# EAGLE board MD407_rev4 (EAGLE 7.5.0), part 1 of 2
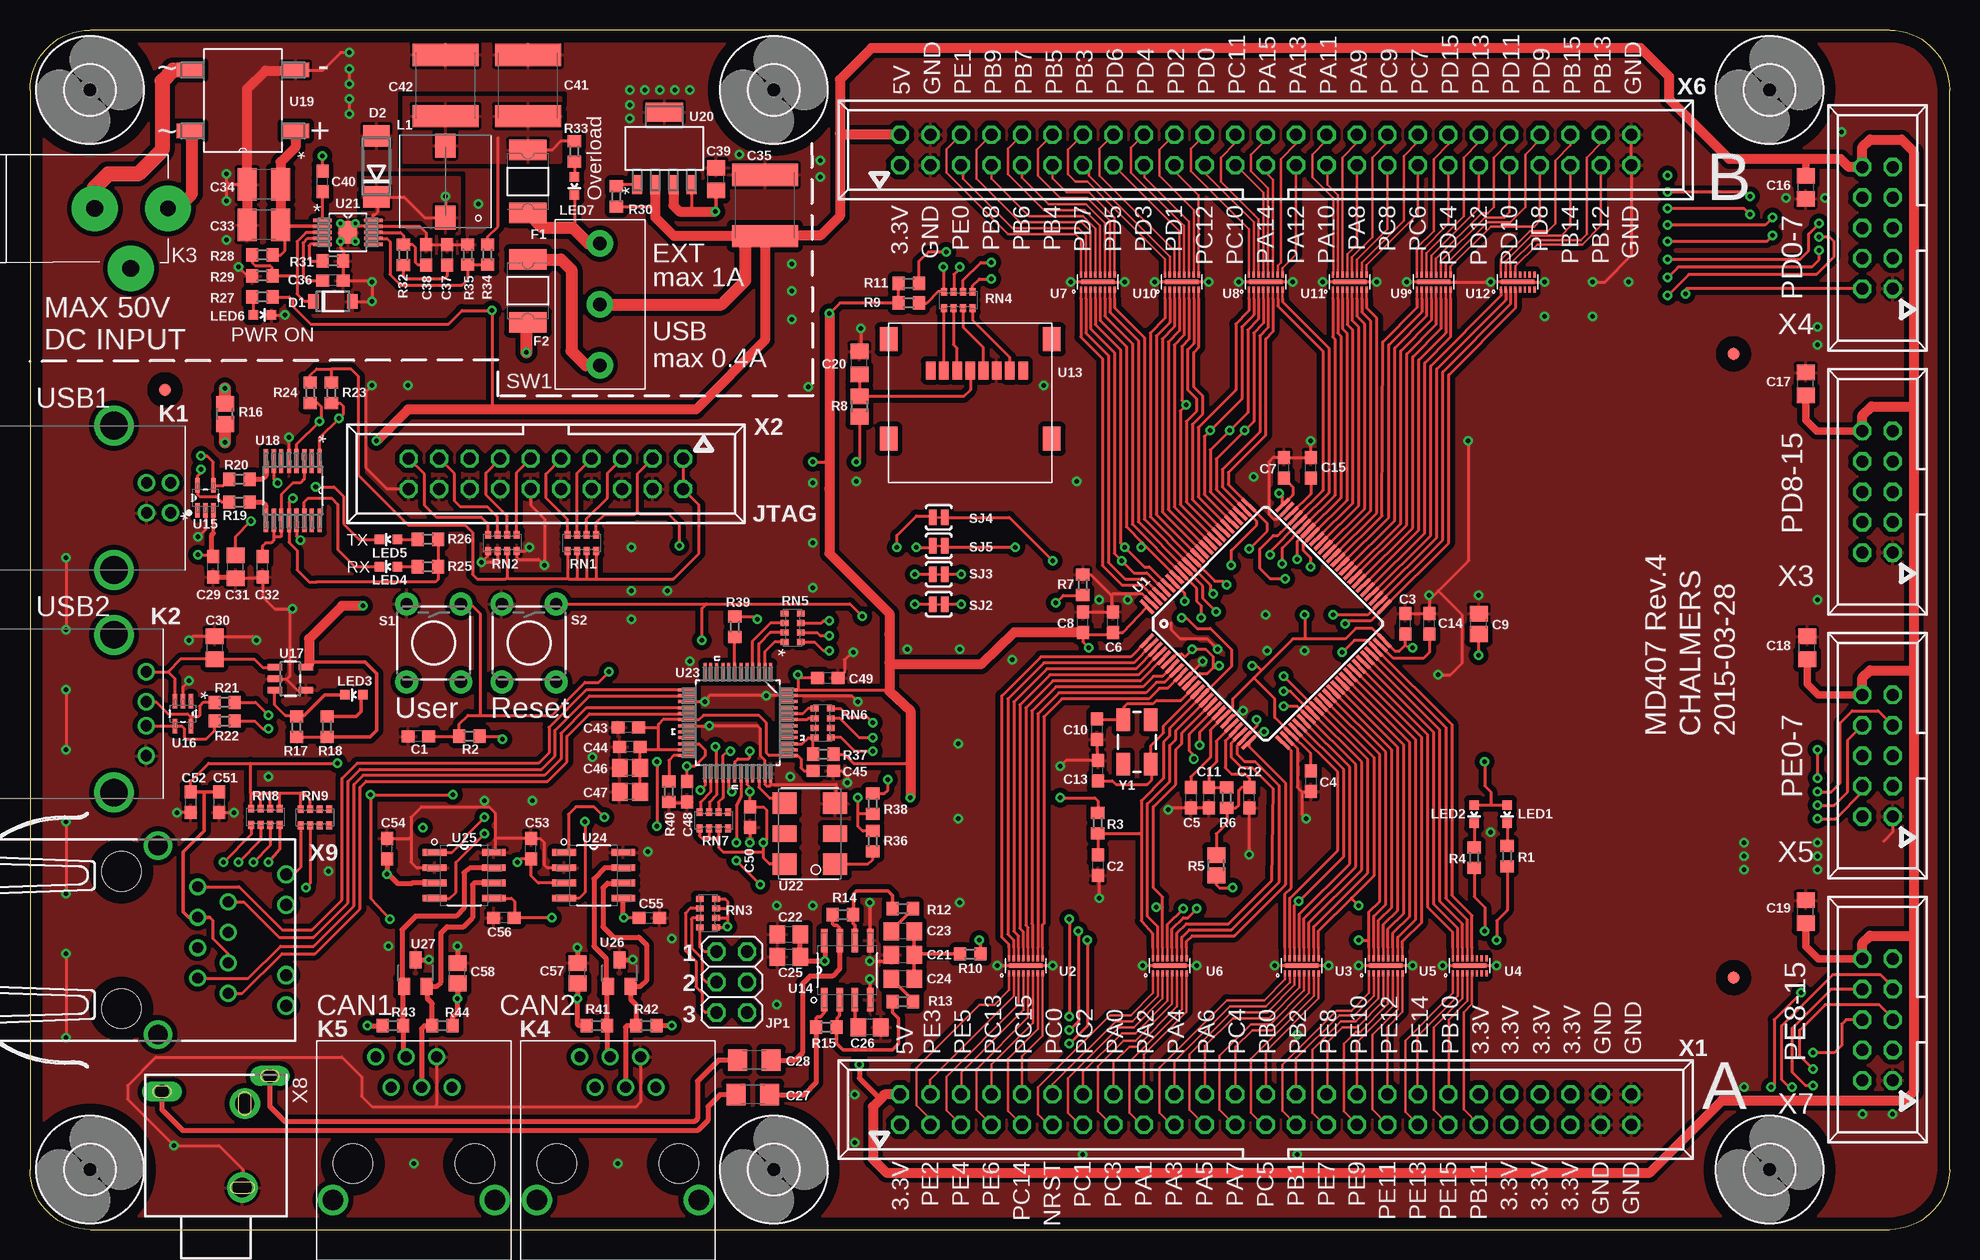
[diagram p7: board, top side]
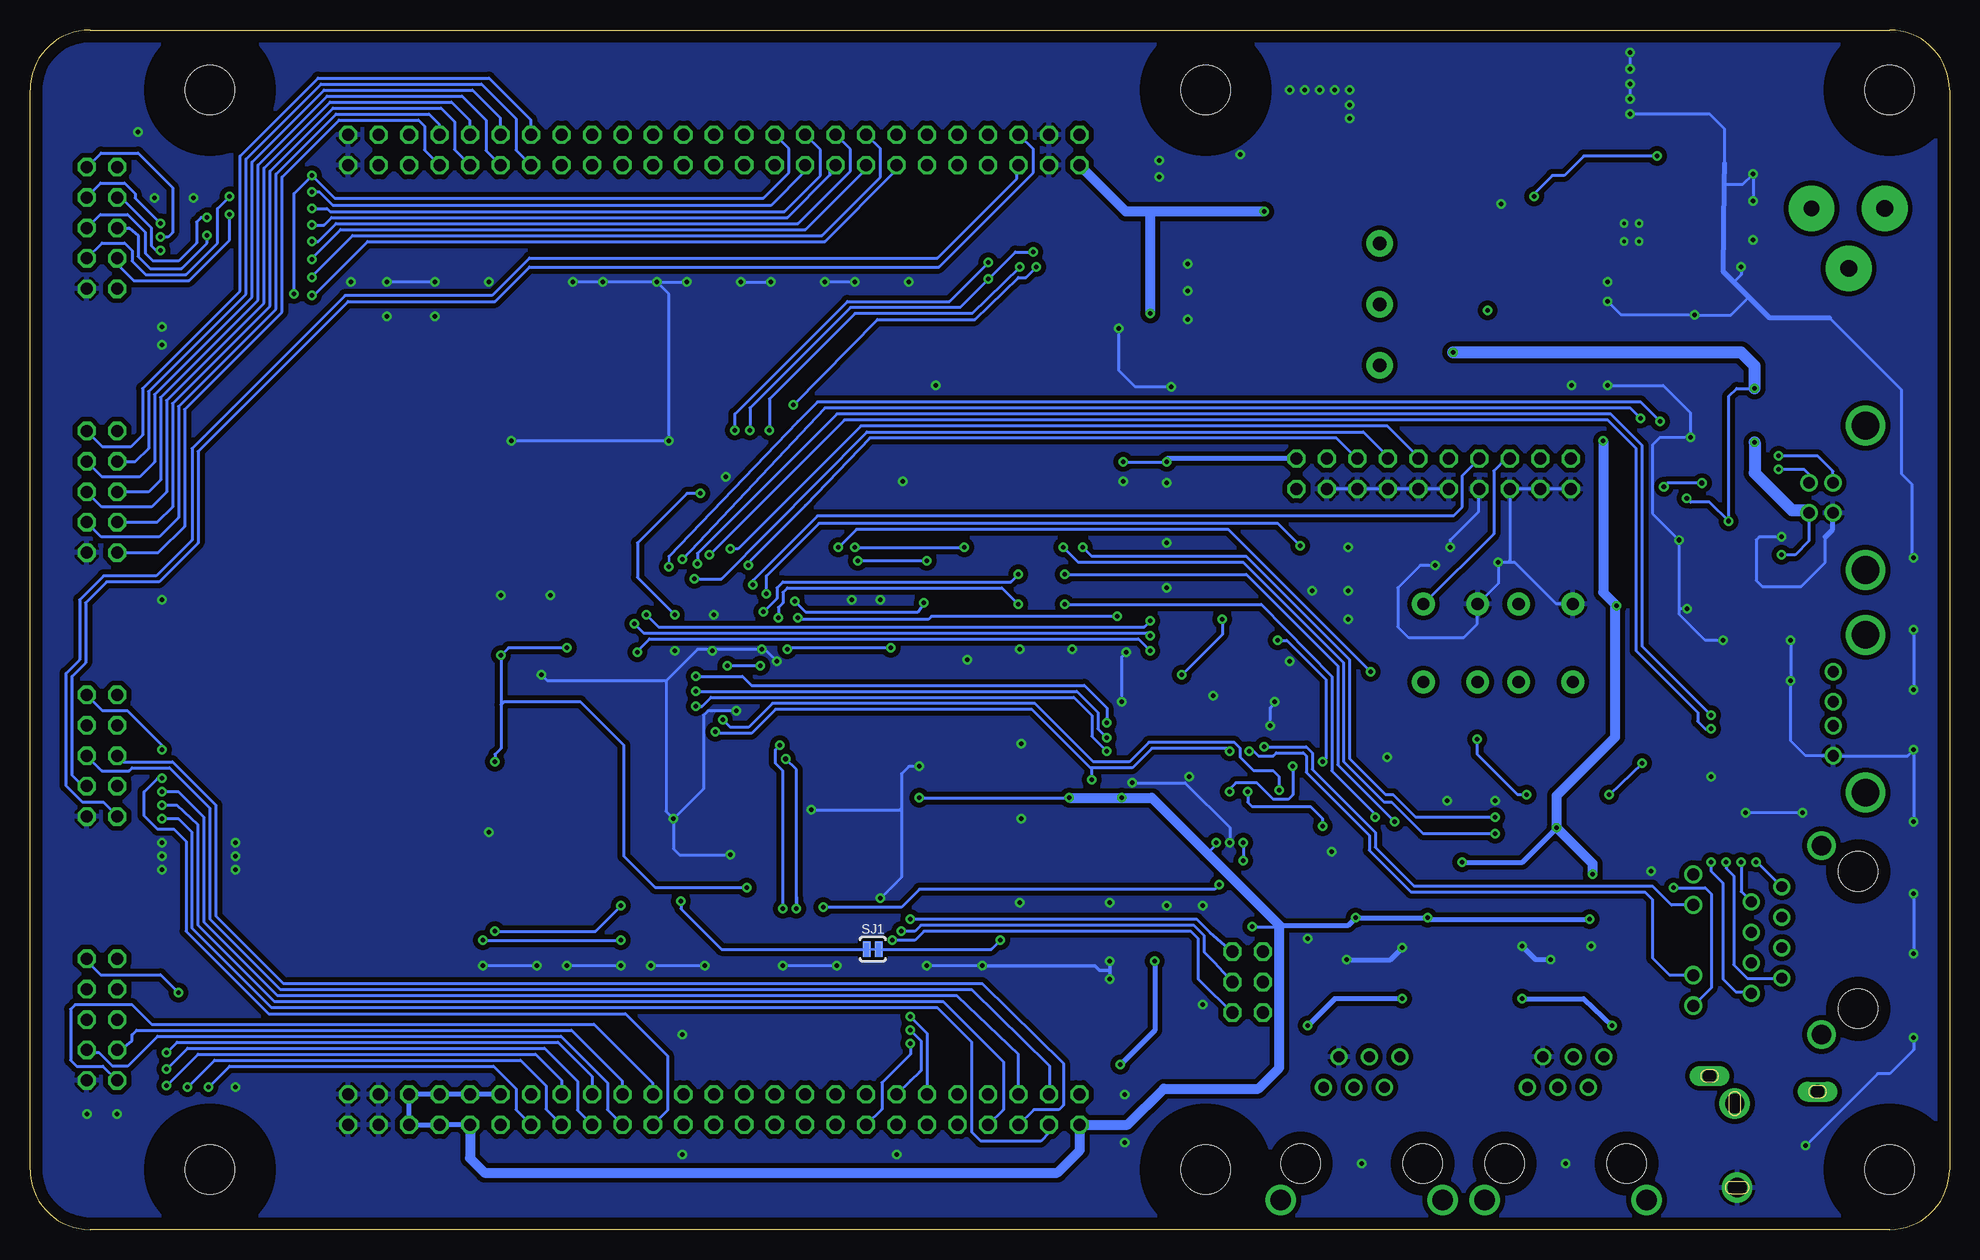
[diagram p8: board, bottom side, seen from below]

Size 160 x 100 mm. Coordinates in mm from the lower left corner, seen from the top.
Outline: 5,0 155,0 arc90 160,5 160,95 arc90 155,100 5,100 arc90 0,95 0,5 arc90 5,0
Copper layers (1*16): Top 0.035mm / dielectric 1.5mm / Bottom 0.035mm
Design rules "default *": minimum track width 0.2mm, minimum drill 0.3mm, track to track 5mil, track to pad 3mil, pad to pad 3mil, via to via 8mil, smd to smd 4mil, copper to edge 40mil, drill to drill 8mil, minimum pad ring 10mil, minimum via ring 8mil, stop-mask expansion 1mil, vias tented up to drill 16mil, thermal gap 10mil
Net classes: 1 HP: width 0.762 mm

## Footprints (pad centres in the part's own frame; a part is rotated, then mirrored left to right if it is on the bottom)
C0603 = smd 1.1 x 1: 1 -0.85,0; 2 0.85,0
C0805 = smd 1.3 x 1.5: 1 -0.85,0; 2 0.85,0
C0805' = smd 1.3 x 1.5: 1 -0.95,0; 2 0.95,0
C1206 = smd 1.6 x 1.8: 1 -1.4,0; 2 1.4,0
C1210 = smd 1.6 x 2.7: 1 -1.4,0; 2 1.4,0
C2220K = smd 1.85 x 5.5: 1 -2.55,0; 2 2.55,0
SOD123FL = smd 0.91 x 1.22: A 1.625,0; C -1.625,0
DO214AA = smd 1.8 x 2.2: A 2.55,0; C -2.55,0
PTC1812L = smd 1.7 x 3.15: 1 -2.62,0; 2 2.62,0
4,1 = hole 4.1: 0,0
2X03 = drill 1.016 octagon: 1 -2.54,-1.27; 2 -2.54,1.27; 3 0,-1.27; 4 0,1.27; 5 2.54,-1.27; 6 2.54,1.27
61400416121 = drill 0.92: 1 1.25,4.71; 2 -1.25,4.71; 3 -1.25,2.71; 4 1.25,2.71 | drill 2.3: Z1 -6.02,0; Z2 6.02,0
61400416021 = drill 0.92: 1 -3.5,2.7; 2 -1,2.7; 3 1,2.7; 4 3.5,2.7 | drill 2.3: 5 -6.57,0; 6 6.57,0
DC-PLUG = drill 1.3 pad 3.81: 1 0,0 | drill 1.4 pad 3.81: 2 3.1,5; 3 6.1,0
615006143421 = drill 0.9: 1 -3.175,8.89; 2 -1.905,6.35; 3 -0.635,8.89; 4 0.635,6.35; 5 1.905,8.89; 6 3.175,6.35 | drill 1.7: Z1 -6.75,-3.05; Z2 6.75,-3.05 | hole 3.25: -5.08,0; 5.08,0
WE-PD_7332/7345_PLASTIC_BASE = smd 1.7 x 2: 1 0,3; 2 0,-3
LED-0603 = smd 0.8 x 0.8: A 0,-0.75; C 0,0.75
R0603 = smd 1 x 1.1: 1 -0.85,0; 2 0.85,0
R0805 = smd 1.3 x 1.5: 1 -0.85,0; 2 0.85,0
CAY16 = smd 0.5 x 0.65: 1 -1.2,-0.675; 2 -0.4,-0.675; 3 0.4,-0.675; 4 1.2,-0.675; 5 1.2,0.675; 6 0.4,0.675; 7 -0.4,0.675; 8 -1.2,0.675
TACTILE-PTH = drill 1.016 pad 1.88: 1 -3.251,2.261; 2 3.251,2.261; 3 -3.251,-2.261; 4 3.251,-2.261
SJ_2S-TRACE = smd 0.635 x 1.27: 1 -0.508,0; 2 0.508,0
25436N = drill 1.1 pad 2.184: P$1 0,-5.08; P$2 0,0; P$3 0,5.08
LQFP100 = smd 1.5 x 0.3: 1 -8,6; 2 -8,5.5; 3 -8,5; 4 -8,4.5; 5 -8,4; 6 -8,3.5; 7 -8,3; 8 -8,2.5; 9 -8,2; 10 -8,1.5; 11 -8,1; 12 -8,0.5; 13 -8,0; 14 -8,-0.5; 15 -8,-1; 16 -8,-1.5; 17 -8,-2; 18 -8,-2.5; 19 -8,-3; 20 -8,-3.5; 21 -8,-4; 22 -8,-4.5; 23 -8,-5; 24 -8,-5.5; 25 -8,-6; 51 8,-6; 52 8,-5.5; 53 8,-5; 54 8,-4.5; 55 8,-4; 56 8,-3.5; 57 8,-3; 58 8,-2.5; 59 8,-2; 60 8,-1.5; 61 8,-1; 62 8,-0.5; 63 8,0; 64 8,0.5; 65 8,1; 66 8,1.5; 67 8,2; 68 8,2.5; 70 8,3.5; 71 8,4; 72 8,4.5; 73 8,5; 74 8,5.5; 75 8,6 | smd 0.3 x 1.5: 26 -6,-8; 27 -5.5,-8; 28 -5,-8; 29 -4.5,-8; 30 -4,-8; 31 -3.5,-8; 32 -3,-8; 33 -2.5,-8; 34 -2,-8; 35 -1.5,-8; 36 -1,-8; 37 -0.5,-8; 38 0,-8; 39 0.5,-8; 40 1,-8; 41 1.5,-8; 42 2,-8; 43 2.5,-8; 44 3,-8; 45 3.5,-8; 46 4,-8; 47 4.5,-8; 48 5,-8; 49 5.5,-8; 50 6,-8; 76 6,8; 77 5.5,8; 78 5,8; 79 4.5,8; 80 4,8; 81 3.5,8; 82 3,8; 83 2.5,8; 84 2,8; 85 1.5,8; 86 1,8; 87 0.5,8; 88 0,8; 89 -0.5,8; 90 -1,8; 91 -1.5,8; 92 -2,8; 93 -2.5,8; 94 -3,8; 95 -3.5,8; 96 -4,8; 97 -4.5,8; 98 -5,8; 99 -5.5,8; 100 -6,8 | smd 1.5 x 0.35: 69 8,3
16-WFDFN = smd 0.2 x 0.5: 1 -1.4,-0.625; 2 -1,-0.625; 3 -0.6,-0.625; 4 -0.2,-0.625; 5 0.2,-0.625; 6 0.6,-0.625; 7 1,-0.625; 8 1.4,-0.625; 9 1.4,0.625; 10 1,0.625; 11 0.6,0.625; 12 0.2,0.625; 13 -0.2,0.625; 14 -0.6,0.625; 15 -1,0.625; 16 -1.4,0.625 | smd 2.8 x 0.4: 17 0,0
MICROSD_500901-0801 = smd 0.8 x 1.5: P$1 -3.3,0.75; P$2 -2.2,0.75; P$3 -1.1,0.75; P$4 0,0.75; P$5 1.1,0.75; P$6 2.2,0.75; P$7 3.3,0.75; P$8 4.4,0.75 | smd 1.45 x 2: P$9 -6.8,3.35; P$10 6.8,3.35; P$11 -6.8,-4.95; P$12 6.8,-4.95
SOIC127P600X175-8N = smd 1.981 x 0.559: 1 -2.464,1.905; 2 -2.464,0.635; 3 -2.464,-0.635; 4 -2.464,-1.905; 5 2.464,-1.905; 6 2.464,-0.635; 7 2.464,0.635; 8 2.464,1.905
SOT65P220X110-5N = smd 1.168 x 0.356: 1 -1.041,0.66; 2 -1.041,0; 3 -1.041,-0.66; 4 1.041,-0.66; 5 1.041,0.66
SOT23-5 = smd 0.55 x 1.2: 1 -0.95,-1.3; 2 0,-1.3; 3 0.95,-1.3; 4 0.95,1.3; 5 -0.95,1.3
SOP63P600X175-16N = smd 1.981 x 0.356: 1 -2.464,2.235; 2 -2.464,1.575; 3 -2.464,0.965; 4 -2.464,0.305; 5 -2.464,-0.305; 6 -2.464,-0.965; 7 -2.464,-1.575; 8 -2.464,-2.235; 9 2.464,-2.235; 10 2.464,-1.575; 11 2.464,-0.965; 12 2.464,-0.305; 13 2.464,0.305; 14 2.464,0.965; 15 2.464,1.575; 16 2.464,2.235
SOT508P985X260-4N = smd 2.235 x 1.245: 1 -4.394,2.54; 2 -4.394,-2.54; 3 4.394,-2.54; 4 4.394,2.54
SOT15P696X180-5N = smd 1.6 x 0.838: 1 -3.023,2.261; 2 -3.023,0.762; 3 -3.023,-0.762; 4 -3.023,-2.261 | smd 1.6 x 3.099: 5 3.023,0
SOP50P490X110-11N = smd 1.549 x 0.279: 1 -2.108,0.991; 2 -2.108,0.508; 3 -2.108,0; 4 -2.108,-0.508; 5 -2.108,-0.991; 6 2.108,-0.991; 7 2.108,-0.508; 8 2.108,0; 9 2.108,0.508; 10 2.108,0.991 | smd 1.575 x 1.88: 11 0,0
CRYSTAL-SMD-7.5X5.2-6PIN = smd 1.8 x 2: 1 -2.54,-2.1; 2 2.54,-2.1; 3 2.54,2.1; 4 -2.54,2.1 | smd 1.4 x 2: NC0 0,-2.1; NC1 0,2.1
QFP50P900X900X160-48N = smd 1.473 x 0.254: 1 -4.242,2.743; 2 -4.242,2.261; 3 -4.242,1.753; 4 -4.242,1.245; 5 -4.242,0.762; 6 -4.242,0.254; 7 -4.242,-0.254; 8 -4.242,-0.762; 9 -4.242,-1.245; 10 -4.242,-1.753; 11 -4.242,-2.261; 12 -4.242,-2.743; 25 4.242,-2.743; 26 4.242,-2.261; 27 4.242,-1.753; 28 4.242,-1.245; 29 4.242,-0.762; 30 4.242,-0.254; 31 4.242,0.254; 32 4.242,0.762; 33 4.242,1.245; 34 4.242,1.753; 35 4.242,2.261; 36 4.242,2.743 | smd 0.254 x 1.473: 13 -2.743,-4.242; 14 -2.261,-4.242; 15 -1.753,-4.242; 16 -1.245,-4.242; 17 -0.762,-4.242; 18 -0.254,-4.242; 19 0.254,-4.242; 20 0.762,-4.242; 21 1.245,-4.242; 22 1.753,-4.242; 23 2.261,-4.242; 24 2.743,-4.242; 37 2.743,4.242; 38 2.261,4.242; 39 1.753,4.242; 40 1.245,4.242; 41 0.762,4.242; 42 0.254,4.242; 43 -0.254,4.242; 44 -0.762,4.242; 45 -1.245,4.242; 46 -1.753,4.242; 47 -2.261,4.242; 48 -2.743,4.242
SOT23 = smd 1 x 1.4: 1 -0.95,-1.1; 2 0.95,-1.1; 3 0,1.1
FIDUCIAL_1MM = smd 1 x 1: 1 0,0
057-050-1 = drill 1 octagon: 1 -30.48,-1.27; 2 -30.48,1.27; 3 -27.94,-1.27; 4 -27.94,1.27; 5 -25.4,-1.27; 6 -25.4,1.27; 7 -22.86,-1.27; 8 -22.86,1.27; 9 -20.32,-1.27; 10 -20.32,1.27; 11 -17.78,-1.27; 12 -17.78,1.27; 13 -15.24,-1.27; 14 -15.24,1.27; 15 -12.7,-1.27; 16 -12.7,1.27; 17 -10.16,-1.27; 18 -10.16,1.27; 19 -7.62,-1.27; 20 -7.62,1.27; 21 -5.08,-1.27; 22 -5.08,1.27; 23 -2.54,-1.27; 24 -2.54,1.27; 25 0,-1.27; 26 0,1.27; 27 2.54,-1.27; 28 2.54,1.27; 29 5.08,-1.27; 30 5.08,1.27; 31 7.62,-1.27; 32 7.62,1.27; 33 10.16,-1.27; 34 10.16,1.27; 35 12.7,-1.27; 36 12.7,1.27; 37 15.24,-1.27; 38 15.24,1.27; 39 17.78,-1.27; 40 17.78,1.27; 41 20.32,-1.27; 42 20.32,1.27; 43 22.86,-1.27; 44 22.86,1.27; 45 25.4,-1.27; 46 25.4,1.27; 47 27.94,-1.27; 48 27.94,1.27; 49 30.48,-1.27; 50 30.48,1.27
057-020-1 = drill 1 octagon: 1 -11.43,-1.27; 2 -11.43,1.27; 3 -8.89,-1.27; 4 -8.89,1.27; 5 -6.35,-1.27; 6 -6.35,1.27; 7 -3.81,-1.27; 8 -3.81,1.27; 9 -1.27,-1.27; 10 -1.27,1.27; 11 1.27,-1.27; 12 1.27,1.27; 13 3.81,-1.27; 14 3.81,1.27; 15 6.35,-1.27; 16 6.35,1.27; 17 8.89,-1.27; 18 8.89,1.27; 19 11.43,-1.27; 20 11.43,1.27
057-010-1 = drill 1 octagon: 1 -5.08,-1.27; 2 -5.08,1.27; 3 -2.54,-1.27; 4 -2.54,1.27; 5 0,-1.27; 6 0,1.27; 7 2.54,-1.27; 8 2.54,1.27; 9 5.08,-1.27; 10 5.08,1.27
KLBR4 = drill 1.6 pad 2.54: B -2.4,-3.5; S -2.2,3.5 | drill 1.1 pad 1.2 long: R -4.5,-5.8; T 4.5,-4.5
J1 = drill 0.9 pad 1.3: 1 4.445,2.54; 2 3.175,0; 3 1.905,2.54; 4 0.635,0; 5 -0.635,2.54; 6 -1.905,0; 7 -3.175,2.54; 8 -4.445,0 | drill 1 pad 1.422: 9 5.465,7.37; 10 2.925,7.37; 11 -2.925,7.37; 12 -5.465,7.37 | drill 1.6 pad 2.184: M1 -7.875,-3.3; M2 7.875,-3.3 | hole 3.3: 5.715,-6.35; -5.715,-6.35
CRYSTAL-SMD-5X3 = smd 1.9 x 1.1: 1 -1.85,-1.15; 2 1.85,-1.15; 3 1.85,1.15; 4 -1.85,1.15

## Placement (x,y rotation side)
C1  100n  [C0603]  32.38,41.12 180 top
C2  100n  [C0603]  89,30.38 270 top
C3  100n  [C0603]  114.62,50.5 90 top
C4  100n  [C0603]  106.75,37.38 270 top
C5  100n  [C0603]  96.75,36 270 top
C6  100n  [C0603]  90.25,50.62 90 top
C7  100n  [C0603]  104.5,63.5 90 top
C8  100n  [C0603]  87.75,50.62 90 top
C9  4u7/X7R/16V  [C0805]  120.75,50.5 90 top
C10  22p  [C0603]  88.96,41.72 90 top
C11  2u2/X5R/6V3  [C0603]  98.25,36 270 top
C12  2u2/X5R/6V3  [C0603]  101.62,36 90 top
C13  22p  [C0603]  89,38.25 90 top
C14  2u2/X5R/6V3  [C0603]  116.62,50.5 90 top
C15  2u2/X5R/6V3  [C0603]  106.75,63.5 90 top
C16  4u7/X7R/16V  [C0805']  148,86.88 270 top
C17  4u7/X7R/16V  [C0805']  148,70.5 90 top
C18  4u7/X7R/16V  [C0805']  148.12,48.5 90 top
C19  4u7/X7R/16V  [C0805']  148,26.5 90 top
C20  4u7/X7R/16V  [C0805']  69.12,72.25 90 top
C21  220n/X7R/25V  [C0805']  72.75,22.91 180 top
C22  4u7/X7R/16V  [C0805']  63.25,24.62 0 top
C23  1u/X7R/25V  [C0805']  72.75,24.88 180 top
C24  1u/X7R/25V  [C0805']  72.75,20.91 180 top
C25  4u7/X7R/16V  [C0805']  63.25,22.75 0 top
C26  1u/X7R/25V  [C0805']  69.98,16.87 180 top
C27  22u/X5R/6V3  [C1206]  60.25,11.25 180 top
C28  22u/X5R/6V3  [C1206]  60.38,14.12 180 top
C29  100n  [C0603]  15.25,55.25 90 top
C30  4u7/X7R/16V  [C0805']  15.38,48.5 270 top
C31  4u7/X7R/16V  [C0805']  17.12,55.25 90 top
C32  100n  [C0603]  19.38,55.25 90 top
C33  4u7/X7S/100V  [C1210]  19.5,83.75 180 top
C34  4u7/X7S/100V  [C1210]  19.5,87.12 180 top
C35  47u/X7R/16V  [C2220K]  61.25,85.38 90 top
C36  3n9  [C0603]  25.25,79.12 180 top
C37  2n7  [C0603]  34.75,81.25 270 top
C38  4p7  [C0603]  33,81.25 270 top
C39  4u7/X7R/16V  [C0805']  57.19,87.57 90 top
C40  100n  [C0603]  24.38,87.38 90 top
C41  47u/X7R/16V  [C2220K]  41.5,95.38 90 top
C42  47u/X7R/16V  [C2220K]  34.62,95.38 90 top
C43  100n  [C0603]  49.88,41.88 180 top
C44  100n  [C0603]  50,40.25 180 top
C45  100n  [C0603]  66.12,38.25 0 top
C46  4u7/X7R/16V  [C0805]  50,38.5 180 top
C47  4u7/X7R/16V  [C0805]  50,36.5 180 top
C48  100n  [C0603]  54.75,36.5 270 top
C49  100n  [C0603]  66.5,46 0 top
C50  100n  [C0603]  60,34.38 270 top
C51  100n  [C0603]  15.75,35.62 270 top
C52  100n  [C0603]  13.38,35.62 270 top
C53  100n  [C0603]  41.75,31.75 90 top
C54  100n  [C0603]  29.75,31.75 90 top
C55  100n  [C0603]  51.62,26 0 top
C56  100n  [C0603]  39.5,26 180 top
C57  4.7nF/100V  [C0805]  45.62,21.38 90 top
C58  4.7nF/100V  [C0805]  35.62,21.38 90 top
D1  SMF5.0AT1  [SOD123FL]  25.25,77.38 0 top
D2  SS2H10-E3/52T  [DO214AA]  28.88,88.62 90 top
F1  1A  [PTC1812L]  41.5,87.38 90 top
F2  400mA  [PTC1812L]  41.5,78.25 270 top
H1  MOUNT-HOLE4.1  [4,1]  145,5 0 top
H2  MOUNT-HOLE4.1  [4,1]  5,5 0 top
H3  MOUNT-HOLE4.1  [4,1]  62,5 0 top
H4  MOUNT-HOLE4.1  [4,1]  5,95 0 top
H5  MOUNT-HOLE4.1  [4,1]  62,95 0 top
H6  MOUNT-HOLE4.1  [4,1]  145,95 0 top
JP1  [2X03]  58.5,20.62 270 top
K1  61400416121  [61400416121]  7,61 270 top
K2  61400416021  [61400416021]  7,43 270 top
K3  FC681465P  [DC-PLUG]  11.5,85.12 180 top
K4  615006143421  [615006143421]  49,5.5 0 top
K5  615006143421  [615006143421]  32,5.5 0 top
L1  7447789118  [WE-PD_7332/7345_PLASTIC_BASE]  34.62,87.38 180 top
LED1  RED  [LED-0603]  123.12,34.62 180 top
LED2  Green  [LED-0603]  120.38,34.62 180 top
LED3  RED  [LED-0603]  27,44.58 90 top
LED4  Green  [LED-0603]  29.86,55.26 90 top
LED5  Blue  [LED-0603]  29.86,57.54 90 top
LED6  Green  [LED-0603]  19.38,76.25 270 top
LED7  RED  [LED-0603]  45.38,87 180 top
R1  100R  [R0603]  123.12,31.12 90 top
R2  10k  [R0603]  36.62,41.12 0 top
R3  10k  [R0603]  89,33.88 90 top
R4  100R  [R0603]  120.38,31 90 top
R5  742792097  [R0805]  98.88,30.38 90 top
R6  59R  [R0603]  99.75,36 270 top
R7  75k  [R0603]  87.75,53.75 270 top
R8  742792097  [R0805]  69.12,68.62 270 top
R9  10k  [R0603]  73.25,77.25 180 top
R10  27R  [R0603]  78.38,22.97 180 top
R11  10k  [R0603]  73.25,78.88 180 top
R12  20k  [R0603]  72.75,26.75 180 top
R13  20k  [R0603]  72.75,19 180 top
R14  20k  [R0603]  67.75,26.25 180 top
R15  20k  [R0603]  66.38,16.88 180 top
R16  742792097  [R0805]  16.25,68 90 top
R17  30k  [R0603]  22.23,41.91 270 top
R18  620R  [R0603]  24.77,41.91 270 top
R19  27R  [R0603]  17.44,60.64 180 top
R20  27R  [R0603]  17.44,62.55 180 top
R21  27R  [R0603]  16.23,43.95 180 top
R22  27R  [R0603]  16.23,42.39 180 top
R23  10k  [R0603]  25.12,69.75 90 top
R24  10k  [R0603]  23.36,69.77 90 top
R25  620R  [R0603]  33.16,55.26 0 top
R26  620R  [R0603]  33.16,57.54 0 top
R27  620R  [R0603]  19.38,77.75 0 top
R28  dnm  [R0603]  19.38,81.25 0 top
R29  dnm  [R0603]  19.38,79.5 0 top
R30  10k  [R0603]  48.88,86.12 270 top
R31  200k  [R0603]  25.25,80.75 180 top
R32  75k  [R0603]  31.12,81.25 90 top
R33  620R  [R0603]  45.38,89.88 270 top
R34  30k  [R0603]  38.14,81.28 90 top
R35  5k6  [R0603]  36.49,81.28 270 top
R36  2k2  [R0603]  70.25,32.38 90 top
R37  1k5  [R0603]  66.12,39.62 180 top
R38  1k5  [R0603]  70.25,35.5 90 top
R39  2k2  [R0603]  58.75,50.25 270 top
R40  4.87k  [R0603]  53.25,36.5 90 top
R41  59R  [R0603]  47.25,17 0 top
R42  59R  [R0603]  51.38,17 0 top
R43  59R  [R0603]  30.25,17 0 top
R44  59R  [R0603]  34.38,17 0 top
RN1  10k  [CAY16]  46,57.25 180 top
RN2  10k  [CAY16]  39.38,57.25 180 top
RN3  10k  [CAY16]  56.5,26.38 90 top
RN4  27R  [CAY16]  77.38,77.5 0 top
RN5  51R  [CAY16]  63.58,50.17 90 top
RN6  51R  [CAY16]  66.08,42.23 90 top
RN7  2k2  [CAY16]  57,34.12 180 top
RN8  51R  [CAY16]  19.62,34.41 180 top
RN9  330R  [CAY16]  23.75,34.38 0 top
S1  SKQBARA010PTH  [TACTILE-PTH]  33.66,48.9 270 top
S2  SKQBARA010PTH  [TACTILE-PTH]  41.59,48.9 270 top
SJ1  SOLDERJUMPERTRACE  [SJ_2S-TRACE]  89.75,23.38 0 bottom
SJ2  SOLDERJUMPERTRACE  [SJ_2S-TRACE]  75.75,52.12 180 top
SJ3  SOLDERJUMPERTRACE  [SJ_2S-TRACE]  75.75,54.62 180 top
SJ4  SOLDERJUMPERTRACE  [SJ_2S-TRACE]  75.75,59.38 180 top
SJ5  SOLDERJUMPERTRACE  [SJ_2S-TRACE]  75.75,57 180 top
SW1  25436NAH  [25436N]  47.5,77.12 0 top
U1  STM32F407VGT7  [LQFP100]  103,50.5 45 top
U2  TPD8F003  [16-WFDFN]  83,22 0 top
U3  TPD8F003  [16-WFDFN]  106,22 0 top
U4  TPD8F003  [16-WFDFN]  120,22 0 top
U5  TPD8F003  [16-WFDFN]  113,22 0 top
U6  TPD8F003  [16-WFDFN]  95,22 0 top
U7  TPD8F003  [16-WFDFN]  89,79 0 top
U8  TPD8F003  [16-WFDFN]  103,79 0 top
U9  TPD8F003  [16-WFDFN]  117,79 0 top
U10  TPD8F003  [16-WFDFN]  96,79 0 top
U11  TPD8F003  [16-WFDFN]  110,79 0 top
U12  TPD8F003  [16-WFDFN]  124,79 0 top
U13  500901-0801  [MICROSD_500901-0801]  78.38,70.88 0 top
U14  TPA6111A2D  [SOIC127P600X175-8N]  68.12,21.62 90 top
U15  SP3003-02JTG  [SOT65P220X110-5N]  14.62,61 90 top
U16  SP3003-02JTG  [SOT65P220X110-5N]  12.75,43 270 top
U17  STMPS2141STR  [SOT23-5]  21.71,45.91 270 top
U18  FT230XS  [SOP63P600X175-16N]  21.91,61.59 270 top
U19  DF01S  [SOT508P985X260-4N]  17.75,94.12 180 top
U20  LP3875EMP-3.3  [SOT15P696X180-5N]  52.88,90.12 90 top
U21  TPS54160ADGQ  [SOP50P490X110-11N]  26.5,83.12 0 top
U22  FXO-HC736R-50  [CRYSTAL-SMD-7.5X5.2-6PIN]  65,33 90 top
U23  DP83848CVV  [QFP50P900X900X160-48N]  59,42.25 270 top
U24  MAX13054ASA+  [SOIC127P600X175-8N]  46.99,29.53 0 top
U25  MAX13054ASA+  [SOIC127P600X175-8N]  36.2,29.53 0 top
U26  PESD2CAN,215  [SOT23]  49.12,21.38 0 top
U27  PESD2CAN,215  [SOT23]  32.12,21.38 0 top
U$1  FIDUCIAL  [FIDUCIAL_1MM]  11.25,70 0 top
U$2  FIDUCIAL  [FIDUCIAL_1MM]  142,21 0 top
U$3  FIDUCIAL  [FIDUCIAL_1MM]  142,73 0 top
U$4  [A4L-LOC]  not placed on the board
X1  61205021621  [057-050-1]  103,10 0 top
X2  61202021621  [057-020-1]  43,63 180 top
X3  61201021621  [057-010-1]  154,61.5 90 top
X4  61201021621  [057-010-1]  154,83.5 90 top
X5  61201021621  [057-010-1]  154,39.5 90 top
X6  61205021621  [057-050-1]  103,90 0 top
X7  61201021621  [057-010-1]  154,17.5 90 top
X8  KLBR4  [KLBR4]  15.5,7 180 top
X9  J1011F01PNL  [J1]  13.97,24.13 270 top
Y1  8MHz  [CRYSTAL-SMD-5X3]  92.27,40.65 90 top

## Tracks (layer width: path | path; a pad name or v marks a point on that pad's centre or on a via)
3.3V  (via drill 0.4)
  Top 0.254: X9.3 16.51,22.99 15.25,24.25 15.25,25.75 14.96,26.04 X9.6 | 20,36.38 19.25,36.38 | 19.25,36.38 18.38,36.38 | RN8.3 19.23,36.35 19.25,36.38 | RN8.2 20.02,36.35 20,36.38 | 93.09,51.91 U1.100 91.09,49.77 C6.1 90.22,49.62 87.78,49.62 C8.1 87.75,49 v88.25,48.5 | 114.62,48.75 114.12,48.25 113.75,48.25 112.91,49.09 | 114.62,48.75 C3.1 | 96.64,45.51 U1.11 96.67,45.55 97.5,46.38 98.12,46.38 98.62,46.88 | U1.75 104.41,60.41 | C7.1 105.25,61.9 105.25,61.23 U1.75 | U1.6 94.88,47.32 95.56,48 96,48 96.25,47.75 v96.88,48.38 98,48.38 98.62,47.75 98.62,46.88 | U1.75 104.41,61.09 v104.12,61.38 | C4.1 106.75,39.68 U1.28 105.06,41.37 103.75,42.69 103.75,44.25 102,46 | U23.48 64,44.99 | 64,44.99 71.51,44.99 71.62,44.88 | R39.1 60.4,51.1 v60.62,50.88 | 64,44.99 v64,46.25 64.25,46 C49.1 | 22.5,36.38 22.88,36.38 23.35,35.9 RN9.7 | 22.5,36.38 20.88,36.38 | 20.88,36.38 20,36.38 | 22.5,36.38 22.55,36.33 RN9.8 | RN8.4 18.43,36.33 18.38,36.38 | RN8.1 20.82,36.33 20.88,36.38 | RN7.5 55.8,32.83 56,32.62 56.62,32.62 | 56.62,32.62 57.25,32.62 57.4,32.77 RN7.7 57.4,31.85 57.75,31.5 61.12,31.5 | RN7.6 56.6,32.65 56.62,32.62 | U23.22 55.75,40.5 56.25,40 56.25,39.5 55.38,38.62 v54.75,38.62 C48.1 | 71.65,49.65 71.62,49.62 | 18.38,38.88 14.88,38.88 13.38,37.38 C52.1 | 18.38,38.88 v25.62,38.88 | v30,25.88 28.38,27.62 v28.38,36.25 v35.25,36.25 | 112.91,49.09 111.88,50.12 110.5,50.12 109.62,49.25 106.25,49.25 | 106.25,49.25 105.25,49.25 102.62,46.62 | 102.62,46.62 102,46 | v106.25,51.25 106.25,49.25 | U1.50 112.91,49.09 | 98.62,46.88 99,46.88 v99.12,47 | v101.88,47 102.25,47 102.62,46.62 | v115.25,48.5 114.75,48.62 114.62,48.75 | 25.12,71.75 23.88,71.75 23.36,71.23 R24.2
  Top 0.254: 44.88,54.25 45.5,54.25 | 45.5,54.25 46.38,54.25 | 46.38,54.25 47.12,54.25 | RN1.5 44.8,54.33 44.88,54.25 | RN1.6 45.6,54.35 45.5,54.25 | RN1.7 46.4,54.27 46.38,54.25 | 47.12,54.25 47.2,54.33 RN1.8 | R23.2 25.12,71.75 | 25.12,71.75 26.75,71.75 27.38,71.12 27.38,62.88 31.5,58.75 36.25,58.75 36.88,58.12 36.88,54.62 37.25,54.25 39.67,54.25 39.77,54.35 | 44.88,54.25 39.88,54.25 39.77,54.35 | RN2.7 39.77,54.35 | R2.2 39.12,41.12 v39.38,40.88 | v66.62,76.38 67.5,77.25 R9.2 R11.2 | 102,46 100.25,44.25 100.25,43.5 99.47,42.72 U1.19 98.38,41.63 98.38,39.38 96.75,37.75 C5.1 | v120.75,47.88 C9.1 | 47.12,54.25 53.62,54.25 55.75,56.38 55.75,60.41 X2.2 X2.1 | 40.38,26.02 40.38,27.38 40.13,27.62 U25.5 | 40.38,26.02 C56.1 | 40.38,26.02 43.48,26.02 v43.5,26 | C55.1 v49.5,26 | R8.2 69.12,64.25 v68.88,64 | v65.25,64 66.62,64 | R5.1 98.88,28.75 99.12,28.5 v100.25,28.5 | v85.88,36 88.75,36 89,35.75 R3.2 | U20.4 55.14,84.89 55.12,84.88 | R37.1 67.88,39.62 68.62,38.88 73.38,38.88 | U23.32 59.76,37.11 60,36.88 v60,36.5 C50.1 61.15,35.23 61.38,35 61.38,32.5 v61.12,32.25 61.12,31.5 | U22.4 61.66,30.46 61.12,31 61.12,31.5 | R36.2 69.4,33.23 69,33.62 69,34.62 | 69,34.62 v69,36 | R38.1 69.03,34.65 69,34.62 | v121.25,39 121.25,37 121.75,36.5 121.75,35.38 | 121.75,35.38 LED2.A | LED1.A 121.75,35.38 | RN3.4 57.92,27.57 58.12,27.38 58.12,26.75 | 58.12,26.75 58.12,26 | 58.12,26 v58.12,25.25 58.05,25.18 RN3.1 | RN3.3 58.1,26.77 58.12,26.75 | RN3.2 58.1,25.98 58.12,26 | 18.38,36.38 18.38,38.88
  Top 0.305: 66.61,61.77 66.62,61.75 | C39.1 57.19,84.94 v57.12,84.88 | C52.1 14.62,36.48 | 14.62,36.48 C51.1 | 14.96,26.04 13.21,26.04 12.75,26.5 12.75,31.5 14.5,33.25 14.5,36.35 14.62,36.48
  Top 0.406: U24.5 49.38,27.54 49.38,26.12 v49.5,26
  Top 0.813: v66.62,76.38 66.62,64 66.62,61.75 66.62,56.38 71.62,51.38 71.62,49.62 71.62,47.25 | 71.62,47.25 71.62,44.88 73.38,43.25 73.38,38.88 v73.38,36 | U20.3 53.64,85.36 54.12,84.88 55.12,84.88 v57.12,84.88 | C8.1 82.03,49.77 79.25,47.12 71.75,47.12 71.62,47.25
  Bottom 0.254: v88.25,48.5 96.75,48.5 v96.88,48.38 | v60.62,50.88 60.62,49.62 v64,46.25 | v25.62,38.88 v28.38,36.25 | 43.38,25.88 v43.5,26 | v104.12,61.38 105.25,61.38 109.38,57.25 109.38,54.38 v106.25,51.25 | v85.88,36 v73.38,36 | v99.12,47 v101.88,47 | v35.25,36.25 36,36.25 39.38,39.62 v39.38,40.88 | v115.25,48.5 120.12,48.5 v120.75,47.88 120.75,43.75 | 120.75,43.75 120.75,40.12 121.25,39.62 v121.25,39 | v68.88,64 v65.25,64 | v100.25,28.5 107.88,28.5 110.5,31.12 110.5,40.38 114.12,44 120.5,44 120.75,43.75 | v54.75,38.62 54.75,36.25 55.12,35.88 56.38,35.88 57.75,37.25 59.5,37.25 60,36.75 v60,36.5 | v61.12,32.25 61.12,32.12 61.88,31.38 | v58.12,25.25 56,25.25 55.88,25.12
  Bottom 0.406: v43.5,26 v49.5,26 50.12,25.38 55.88,25.38 | 43.38,25.88 v30,25.88 | X1.41 X1.43 X1.45 X1.46 X1.44 X1.42 X1.40 | X2.1 65.25,64.27 v65.25,64
  Bottom 0.813: v66.62,76.38 66.62,84.88 | v73.38,36 v69,36 66.5,36 61.88,31.38 55.88,25.38 55.88,25.12 55.88,13.5 57.62,11.75 65.5,11.75 68.52,8.73 X1.1 72.5,8.71 72.5,6.62 74.38,4.75 122.12,4.75 123.32,5.95 X1.41 | v57.12,84.88 66.62,84.88 | 66.62,84.88 68.67,84.88 X6.1
5V  (via drill 0.4)
  Top 0.254: R17.2 R18.2 | 66.25,24.12 U14.8 | U24.3 42.36,28.89 41.75,29.5 C53.1 40.9,30.9 v40.62,30.62 | 61.25,82.75 C35.1 | R30.2 52.02,85.28 52.12,85.38 | 23.25,47.1 U17.5 23.46,47.31 | R27.2 21.62,77.75 21.88,77.5 21.88,77 23.38,75.5 34.88,75.5 36,76.62 v38.5,76.62 38.5,68.62 38.75,68.38 | 146.25,89 146.5,89.25
  Top 0.305: R18.2 28.36,41.06 28.89,41.59 28.89,46.35 27.94,47.31 23.46,47.31
  Top 0.406: U25.3 31.86,28.89 31.84,28.88 30.62,28.88 29.88,29.62 v29.75,29.62 C54.1 | 66.25,24.12 v66.25,22.38 64.33,22.38 C25.2 C22.2 | v69.12,13.75 69.12,12.62 70.88,10.88
  Top 0.61: X7.10 149.04,22.58 148,23.62 C19.1 | C18.1 148.12,45.5 149.04,44.58 X5.10 | C17.1 148,67.5 148.92,66.58 X3.10 | C16.1 148,89.25
  Top 0.813: v28.88,65.75 31.5,68.38 38.75,68.38 55.5,68.38 61.25,74.13 61.25,82.75 | v27.75,52 26,52 23.25,49.25 23.25,47.1 | 67.5,91.38 67.5,95.88 70.12,98.5 134.25,98.5 136.62,96.12 136.62,94.25 141.62,89.25 146.5,89.25 148,89.25 150.94,89.25 151.6,88.58 X4.10 152.73,90.23 153.38,90.88 156,90.88 157,89.88 157,68.62 | 67.5,91.38 67.5,84.5 65.88,82.88 61.3,82.88 C35.1 59.75,82.83 53.67,82.83 52.12,84.38 52.12,85.38 52.12,87.09 U20.2 | X1.2 71.27,11.27 70.88,10.88 70.25,10.25 70.25,5.88 71.38,4.75 135,4.75 141,10.75 156.25,10.75 157,11.5 157,24.5 | X6.2 67.61,91.27 67.5,91.38 | 157,68.62 157,46.62 | 157,46.62 157,24.5 | X7.10 152.73,23.86 153.38,24.5 157,24.5 | X5.10 152.73,45.98 153.38,46.62 157,46.62 | X3.10 152.73,67.86 153.5,68.62 157,68.62
  Top 1.016: 59.75,82.83 59.62,82.7 59.62,79.12 57.62,77.12 SW1.P$2
  Bottom 0.406: v40.62,30.62 35.62,30.62 v32.75,33.5 | v66.25,22.38 66.25,16.62 v69.12,13.75
  Bottom 0.813: v28.88,65.75 28.88,53.12 v27.75,52 27.88,51.88 27.88,41.06 32.75,36.19 v32.75,33.5 29.75,30.5 v29.75,29.62
GND  (via drill 0.3, 0.4)
  Top 0.254: U18.13 22.21,57.8 v22.54,57.47 | U18.5 21.6,66.03 v21.59,66.04 | U1.27 104.8,40.95 105.62,40.12 105.62,36.88 106,36.5 | U1.74 103.97,59.25 103.62,59.25 103.25,59.62 103.25,64 103.6,64.35 C7.2 C15.2 v106.75,65.75 | 106,36.5 106.72,36.5 C4.2 | U23.19 v56.62,42 60.62,42 60.88,41.75 60.88,39.5 61.26,39.11 U23.35 61.26,37.11 61.38,37 61.62,37 61.75,37.12 | U23.15 v56.25,44 56.64,44.51 U23.47 68.49,44.51 v69,44 | 61.75,37.12 U23.36 | U22.2 67.2,35.64 67.2,37.12 61.75,37.12 | R40.1 52.85,35.55 54.65,35.55 C48.2 | C3.2 C14.2 116.62,52.5 117.38,53.25 | C10.1 88.96,39.14 C13.2 86.35,39.1 v85.88,38.62 | 21.38,45.88 21.62,46.12 21.62,51.5 v21.88,51.75 | 21.38,45.88 20.45,45.88 | v68.62,48.12 68.5,48.12 67.88,47.5 67.88,46.42 67.45,46 C49.2 | 106,36.5 106,34.62 v106.38,34.25 | v89.12,27.62 89.12,29.4 C2.2 | v119.88,65.75 119.88,55.75 117.38,53.25 | C8.2 C6.2 90.12,51.48 90.12,52.88 | R7.1 88.4,54.6 90.12,52.88 | 90.12,52.88 90.25,53 92.72,53 U1.99 | U1.10 v97.75,47.38 | v99,48.38 98.12,49.25 95.88,49.25 95.12,50 95.12,50.6 | U1.20 99.87,42.37 100.75,43.25 v101.12,43.25 | v117.38,46.25 118.38,46.25 119.38,47.25 119.38,51.25 117.38,53.25 | v69.25,75.12 69.25,73.58 C20.2 | v3,56 v3,50 | v3,45 v3,40 | v3,34 v3,28 | v3,23 v3,16 | U16.2 12.75,45.25 v13.25,45.75 | v13.25,49.12 13.57,49.45 C30.1 18.55,49.45 v18.88,49.12 | 22.29,44.96 21.38,45.88 | v21.88,51.75 21.88,51.88 | v21.88,51.75 20.38,51.75 19.38,52.75 C32.1 19.27,54.3 C31.1 | v41.62,56.88 41.33,56.58 RN2.8 40.58,56.05 40.75,55.88 42.38,55.88 v42.88,55.38 42.88,59.25 41.73,60.4 X2.12 | 17.75,3.55 17.75,3.81 17.75,5 15.75,7 v12,7 8.12,10.88 8.12,12 10.49,14.37 26.01,14.37 27.62,12.75 27.62,11.12 28.5,10.25 33.75,10.25
  Top 0.254: 10.25,39.5 K2.4 | 33.75,10.25 50.5,10.25 50.91,10.65 K4.5 | K5.5 33.91,10.4 33.75,10.25 | 31.75,32.75 31.75,34.38 32.62,35.25 38.25,35.25 38.75,34.75 38.75,32.5 | 31.75,32.75 31.75,30.62 32.21,30.16 U25.2 | v101.62,31.25 C12.1 | C11.2 C5.2 95.03,35.15 v94.88,35 | v86.75,79 U7.17 v91.25,79 | v93.75,79 U10.17 v98.25,79 | v100.75,79 U8.17 v105.25,79 | v107.75,79 U11.17 v112.25,79 | v114.75,79 U9.17 v121.75,79 U12.17 v126.25,79 | X6.50 X6.49 133.48,81.23 131.25,79 v130.25,79 | RN2.5 38.17,56.17 v37.62,55.62 38.88,55.62 38.98,55.73 RN2.6 | 38.75,32.5 38.75,31.52 U25.8 | C54.2 31.6,32.6 31.75,32.75 | 38.75,32.5 38.85,32.6 C53.2 42.52,32.6 42.88,32.25 42.88,30.38 43.09,30.16 U24.2 | C50.2 v60,32.25 | X2.20 29.77,61.73 28,63.5 28,69.88 v28.5,70.38 | 27.12,83.62 v27.12,83.88 27.37,83.63 U21.9 32.49,83.63 33,83.12 C38.1 C37.1 36.47,82.1 R35.1 | 27.12,83.62 v25.88,82.38 25.88,81.88 26.12,81.62 26.12,80.78 R31.1 C36.1 28.38,79.12 v28.5,79 v28.5,77.38 D1.A | v27.12,82.38 27.12,82.5 U21.11 | v25.88,83.88 25.88,83.75 U21.11 | 27.12,83.62 27,83.62 U21.11 | 16.62,87.12 C34.2 18.12,87.12 | 16.62,87.12 16.38,87.38 v16.38,88 | v16.38,85.75 16.38,86.88 16.62,87.12 | v80.62,22 U2.17 v85.25,22 | v92.75,22 U6.17 v97.25,22 | v103.75,22 U3.17 v108.25,22 | v110.75,22 U5.17 v115.25,22 | v117.75,22 U4.17 v122.25,22 | v26.62,93 v26.62,94.25 | v26.62,95.5 v26.62,96.75 | v26.62,98.12 25.88,98.12 24.38,96.62 22.12,96.62 | R29.1 18.12,79.5 v17.38,80.25 | C52.2 12.28,34.77 v12.25,34.75 | v17,34.75 15.78,34.75 C51.2 | U15.2 14.62,58.38 v14,57.75 | C45.2 67.62,38.25 68.12,37.75 v68.12,37.25 | LED6.C v21.25,76.25 | X5.1 155.27,33.15 154.5,32.38
  Top 0.305: 70.03,22.53 v70,22.38 71.52,22.38 C21.2 | v70,20.88 70,19.19 U14.4 | U14.5 69.91,24.09 69.88,24.12 69.88,24.25 70,24.38 v70,27.25
  Top 0.406: U26.3 50.23,22.48 v50.25,22.5 | 45.35,22.5 C57.2 v45.62,23.5 | U27.3 33.23,22.48 v33.25,22.5 | 35.9,22.5 C58.2 v35.62,23.62 | C29.1 17.02,54.4 C31.1 | X8.S 17.75,3.5 17.75,3.81
  Top 0.813: U19.2 22.1,96.62 19.62,96.62 18.1,95.1 C34.2 C33.2
  Bottom 0.254: v56.62,42 56.62,43.5 v56.25,44 | v69,44 69,47.75 v68.62,48.12 | v106.38,34.25 106.38,31.75 105.88,31.25 v101.62,31.25 | v119.88,65.75 v106.75,65.75 106.75,78 v107.75,79 | v101.12,43.25 103.5,43.25 103.88,42.88 103.88,36.75 v106.38,34.25 | 107,45.75 104.38,48.38 v99,48.38 98.75,48.38 v97.75,47.38 | 107,45.75 107,34.88 v106.38,34.25 | 107,45.75 116.88,45.75 v117.38,46.25 | v64.88,70.25 67.88,70.25 69.25,71.62 v69.25,75.12 | 10,76 4,70 4,63 3.12,62.12 3.12,56.12 v3,56 | v3,50 v3,45 | v3,34 v3,40 3.5,39.5 K2.4 12,39.5 13.25,40.75 v13.25,45.75 v13.25,49.12 | v3,28 v3,23 | v3,16 3,15 5,13 6,13 v12,7 | v18.88,49.12 20.38,49.12 22.54,51.29 22.54,51.88 | 22.54,51.88 v22.54,57.47 24.77,59.69 24.77,65.41 24.13,66.04 v21.59,66.04 21.62,66.08 21.62,68.12 23.88,70.38 v28.5,70.38 | v21.88,51.75 22.42,51.75 22.54,51.88 | v41.62,56.88 41.62,57.5 39.25,59.88 39.25,61.67 X2.14 | X2.20 X2.18 X2.16 36.65,55.77 36.5,55.62 | X2.12 X2.10 X2.8 X2.6 X2.4 | S1.3 32.77,52.15 36.25,55.62 36.5,55.62 | 36.5,55.62 v37.62,55.62 37.62,53.85 S2.3 39.38,52.1 39.38,50.5 40.5,49.38 45.12,49.38 46,50.25 46,53.5 44.12,55.38 v42.88,55.38 | v68.12,37.25 63.73,37.25 C50.2 v60,32.25 | v16.38,85.75 v16.38,88 17.24,87.13 18.77,87.13 | v80.62,22 v85.25,22 | v92.75,22 v97.25,22 | v103.75,22 v108.25,22 | v110.75,22 v115.25,22 | v117.75,22 v122.25,22 | 18.75,88.88 18.75,91.75 20,93 v26.62,93 | v26.62,94.25 v26.62,95.5 | v26.62,96.75 v26.62,98.12 | v85.88,38.62 86.75,38.62 87.38,38 87.38,35.12 | 87.38,35.12 87.38,29.38 v89.12,27.62 | v94.88,35 87.5,35 87.38,35.12 | v17.38,80.25 17.38,79.62 18,79 | v12.25,34.75 v17,34.75 | v107.75,79 v112.25,79 v114.75,79
  Bottom 0.254: v107.75,79 v105.25,79 | v100.75,79 v98.25,79 | v91.25,79 v93.75,79 | v126.25,79 v130.25,79 | v14,57.75 15.88,57.75 16.12,57.5 16.12,54.12 15.62,53.62 12.38,53.62 10.38,55.62 10.38,57.75 | 16.75,77.75 18.25,76.25 v21.25,76.25 27.38,76.25 v28.5,77.38
  Bottom 0.305: v70,22.38 70,21.62 | 70,21.62 v70,20.88 | v80.62,22 71.25,22 70.88,21.62 70,21.62
  Bottom 0.406: 10,76 15,76 16.75,77.75 18,79 18.88,79.88 18.77,87.13 18.75,88.88 | 10.38,57.75 9.75,58.38 9.75,59.71 K1.4 | v33.25,22.5 34.5,22.5 v35.62,23.62 | v50.25,22.5 46.62,22.5 v45.62,23.5
  other vias: 50,95 51.25,95 52.5,95 53.75,95 55,95 50,93.75 50,92.62 77.38,34.25 77.38,40.5 121.75,33.12 51.5,31.5 46.88,39.38 133.25,79 87.25,62.38 68.88,62.38 61.38,44.5 102,62.75 103,51.25 91.5,52.5 89.12,52.5 103.12,48.25 106.25,48.25 63.38,37.75 50.12,56.88 77.5,27.25 65.25,27 29.88,23.62 37.88,35.75 77.5,48.38 149,52.5 37.38,85.5 59.12,89.62 65.88,89.12 84.5,70.38 50.12,53.25 53.12,53.25 63.5,80.5 63.5,78.25 63.5,75.88 19.88,37.75 24.88,29.88 130.25,76.12 126.25,76.12 81.88,47.5 73.12,48.38 146.38,86 142.88,30 142.88,31.12 142.88,32.25 149.62,86 149,32.25 149,31.12 149,30 142.88,11.88 116.62,52.88 149,73.75 149,75.25 152.75,9.62 155.25,9.62 68.75,11.25 68.75,7.25 32,5.5 49,5.5 65.88,87.75 16.38,82.5 55,47.38 50.12,50.88 65.25,62.25 41.88,35.75 53.5,24.25 62.25,18.75 62.25,27 151,91.5 120.75,52.88 31.5,70.38 87.75,6.25 105.62,6.25 105.62,16.25 65.25,57.25 65.25,53.5
  pour Top (isolate 0.406, rank 3): -12.48,113.99 -28.63,122.52 21.09,116.22 161.29,101.6 161.29,-1.27 -10.83,-2.65
  pour Bottom (isolate 0.406): -5.97,148.15 -18.5,-2 159.25,-4.38 161.88,102.12
N$1
  Top 0.254: R33.2 LED7.A
N$2
  Top 0.406: U18.9 19.67,60.34 19.37,60.64 R19.1
N$3
  Top 0.254: LED6.A 18.62,77.65 R27.1
N$4
  Top 0.254: C38.2 32.35,80.4 32.12,80.62 32.12,81.88 31.88,82.12 31.15,82.12 R32.2 31.12,82.88 30.88,83.12 U21.8
N$5
  Top 0.254: LED4.A R25.1
N$6
  Top 1.016: U19.3 11.94,96.67 11.93,96.67 | 5.38,86.88 5.38,85.15 K3.3
  Top 1.27: 11.93,96.67 11,95.75 11,90 9,88 6.5,88 5.38,86.88
N$7
  Top 0.254: U21.3 23,83.12 22.25,82.38 22.25,79.5 | 22.25,79.5 22.25,78 22.88,77.38 D1.C | 22.25,79.5 R29.2 20.12,79.6 20.12,80.25 20,80.38 18.75,80.38 18.52,80.6 R28.1
N$8
  Top 0.254: RN3.8 55.83,23.55 56.21,23.16 JP1.1
N$9
  Top 0.254: LED2.C R4.2
N$10
  Top 0.254: U20.1 49,87.1 R30.1
N$11  (via drill 0.4)
  Top 0.254: 95.22,54.03 U1.94 96.25,53.01 v96.25,52.38 | v85.5,52.25 86.12,52.88 87.72,52.88 R7.2
  Bottom 0.254: v85.5,52.25 86,51.5 95.38,51.5 v96.25,52.38
N$12
  Top 0.254: U23.24 53.63,39.51 53.25,39.12 R40.2
N$13
  Top 0.406: U18.8 19.67,62.85 19.37,62.55 R20.1
N$14
  Top 0.254: U23.23 52.38,39.99 | 52.38,39.99 51.11,39.99 C44.1 C46.1 C47.1 | 52.38,39.99 52.38,41.88 | 52.38,41.88 52.38,42.12 52.75,42.5 U23.18 55.75,42.5 56.12,42.88 60.75,42.88 61.38,42.25 61.38,39.75 61.62,39.51 U23.37 | U23.37 63.62,39.5 64,39.5 64.25,39.25 64.25,38.5 64.5,38.25 C45.1 | C43.1 52.38,41.88 | U23.37
N$15
  Top 0.254: LED5.A R26.1
N$16  (via drill 0.4)
  Top 0.254: R19.2 15.98,60.64 15.5,61.12 14.12,61.12 13.96,61.28 U15.5 13.96,62.84 14.25,63.12 v14.25,63.38
  Bottom 0.254: K1.2 11.71,62.96 12.12,63.38 v14.25,63.38
N$17
  Top 0.254: U18.14 22.87,60.66 23.18,60.96 25.15,60.96 25.65,60.45 25.65,56.67 27.07,55.26 LED4.C
N$18
  Top 0.254: 13.38,42.75 13.12,43 11.5,43 10.5,44 K2.2 | 13.38,42.75 13.38,41.99 U16.5 | R21.2 14.45,43.95 14.12,43.62 14.12,42.88 14,42.75 13.38,42.75
N$19
  Top 0.254: K2.3 12.05,42 U16.4 12.67,41.96 12.88,41.75 12.88,41 13,40.88 14.62,40.88 15.38,41.62 R22.2
N$20  (via drill 0.4)
  Top 0.254: 16.5,62.64 R20.2 16.09,62.04 U15.4 15.29,63.97 14.75,64.5 v14.25,64.5
  Bottom 0.254: K1.3 9.71,63.21 11,64.5 v14.25,64.5
N$21
  Top 0.305: R18.1 27.2,42.76 27.62,43.18 27.62,44.45 LED3.A
N$22  (via drill 0.4)
  Top 0.254: U18.7 20.33,62.53 v20.64,62.23 | v23.81,61.91 25.34,61.91 26.16,61.09 26.16,58.81 27.44,57.54 LED5.C
  Bottom 0.254: v20.64,62.23 23.5,62.23 v23.81,61.91
N$23
  Top 0.254: RN3.7 55.23,25.98 55.12,25.88 55.12,23.5 56,22.62 56,21 56.38,20.62 JP1.3
N$24
  Top 0.254: R17.1 22.12,42.86 21.27,42.86 20.41,43.72 U17.3
  Top 0.305: LED3.C 24.58,44.58 22.86,42.86 22.33,42.86 R17.1
N$25
  Top 0.305: U14.1 66.22,18.09 65.88,17.75 65.62,17.75 65.5,17.62 65.5,16.9 R15.2
  Top 0.406: C27.1 64.5,11.25 65.53,12.28 R15.2
N$26
  Top 0.406: U24.6 49.44,28.88 48.12,28.88 47.75,28.5 47.75,25.25 48.62,24.38 50.75,24.38 51.38,23.75 51.38,20.75 50.9,20.27 U26.2 50.08,19.18 50.5,18.75 50.5,17.02 R42.1 49.75,17 49.62,16.88 K4.4
N$27
  Top 0.254: C15.1 106.75,61.32 U1.73
N$28
  Top 0.254: U18.3 22.87,62.56 22.54,62.23 21.91,62.23 20.95,61.28 20.95,59.14 U18.11 20.94,57.82 20.88,57.75 20.33,57.75 | U18.10 20.33,57.75 | 20.33,57.75 20.33,57.46 20.12,57.25 19.62,57.25 19.38,57 C32.2
  Top 0.406: 22.86,64.05 U18.3
N$29
  Top 0.406: U24.7 47.91,30.16 47,29.25 47,23.62 48,22.62 48,20.45 U26.1 48.1,20.2 R41.2 48.1,14.65 K4.3
N$30
  Top 0.254: K2.1 11.5,46.5 | 11.5,46.5 12.55,47.55 C30.2 18.7,47.55 19.38,46.88 U17.1 | U16.3 12.09,45.91 11.5,46.5
N$31
  Top 0.254: C37.2 34.75,79.5 34.5,79.25 31.38,79.25 31.12,79.5 R32.1
N$32
  Top 0.254: U23.43 64.18,42.5 64.75,42.5 64.88,42.62 RN6.6
N$33
  Top 0.254: U23.2 61.26,48.18 62.05,48.97 RN5.8
N$34
  Top 0.254: U21.7 29.76,82.62 30,82.38 30,79.62 30.88,78.75 36,78.75 36.5,79.25 36.5,80.42 R35.2 R34.1
N$35
  Top 0.254: U21.1 24.39,86.46 C40.1
N$36
  Top 0.254: R28.2 20.88,81.25 21.25,81.62 21.25,83.4 C33.1
  Top 0.305: C33.1 21.39,83.63 U21.2
  Top 0.813: 22.12,91.57 22.12,90.25 20.88,89 20.88,87.15 C34.1 C33.1
  Top 1.016: 22.12,91.57 U19.1
N$37
  Top 0.254: U23.44 64.43,43.01 64.84,43.42 RN6.5
N$38
  Top 1.016: U19.4 13.5,91.44 13.5,86.38 12.21,85.09 11.54,85.09 K3.1
N$39
  Top 0.254: RN6.8 65.15,41.02 | U23.39 64.37,40.5 64.88,41 65.38,41 RN6.8 | R37.2 65.28,40.9 RN6.8
N$40
  Top 0.254: C20.1 R8.1 77.85,69.47 78.38,70 U13.P$4
N$41
  Top 0.254: RN3.6 55.02,26.77 54.62,26.38 54.62,23.25 55.5,22.38 55.5,20.25 56,19.75 56,18.38 56.29,18.09 JP1.5
N$42
  Top 0.305: U14.6 68.76,25.36 68.6,25.52 R14.1 68.62,26.27 68.62,28 68.88,28.25 71.5,28.25 71.9,27.85 R12.2
N$43
  Top 0.254: U1.22 99.62,40.75 99.62,38.5 100.12,38 101.25,38 101.62,37.62 C12.2 100.97,36.85 100.75,36.62 100.75,35.38 100.53,35.15 R6.2 99.75,33.88 98.88,33 R5.2
N$44
  Top 0.254: U13.P$2 RN4.1
N$45
  Top 0.254: U1.12 95.92,44.12 93.91,44.12 93.6,43.81 91.44,43.81 91.19,43.56 91.19,42.56 Y1.3 89.02,42.5 C10.2
N$46
  Top 0.254: RN4.2 76.97,73.78 77.28,73.47 U13.P$3
N$47
  Top 0.254: U21.4 23.12,82.62 22.75,82.25 22.75,79.5 23.12,79.12 C36.2
N$48  (via drill 0.4)
  Top 0.305: R10.1 79.22,24.02 v79.12,24.12
  Bottom 0.254: SJ1.2 79.88,23.38 v79.12,24.12
N$49
  Top 0.254: U1.13 94.49,41.99 94.49,41.4 93.42,40.34 Y1.1 93.5,38.72 93.5,37.5 93.12,37.12 90.5,37.12 90.22,37.4 C13.1
N$50  (via drill 0.4)
  Top 0.254: RN9.2 23.35,28.85 v23,28.5
  Bottom 0.254: v23,28.5 20.38,28.5 19.88,28 19.88,20.13 X9.9
N$51
  Top 0.254: U23.3 60.75,48.81 61.7,49.77 RN5.7
N$52
  Top 0.254: U23.4 60.24,49.07 61.74,50.57 RN5.6
N$53  (via drill 0.4)
  Top 0.254: X9.1 17.68,19.68 21,23 23.75,23 27.5,26.75 27.5,36.88 28,37.38 43.12,37.38 44.75,39 44.75,41.12 46.62,43 54.75,43 U23.17 | RN8.8 20.82,31.7 v19.88,30.62
  Bottom 0.254: X9.1 16.64,19.81 17.81,19.81 18.88,20.88 18.88,28.88 19.88,29.88 v19.88,30.62
N$54  (via drill 0.4)
  Top 0.254: X9.2 18.2,20.95 20.88,23.62 23.62,23.62 27,27 27,37.12 27.75,37.88 42.88,37.88 44.25,39.25 44.25,41.38 46.37,43.49 U23.16 | RN8.7 20.02,32.02 v18.62,30.62
  Bottom 0.254: X9.2 16.88,20.95 18,22.08 18,29.5 18.62,30.12 v18.62,30.62
N$55
  Top 0.254: U23.7 R39.2
N$56
  Top 0.254: U21.5 23.38,82.13 23.25,82 23.25,80.88 23.38,80.75 R31.2
N$57  (via drill 0.4)
  Top 0.254: RN7.2 57.38,34.82 57.38,35.63 57.75,36 U23.28 57.76,39.51 58.12,39.88 v58.38,39.88
  Bottom 0.254: X9.10 23.33,21.2 24.75,22.62 24.75,27.5 25.38,28.12 44.88,28.12 48.38,31.62 48.38,32.88 53.62,38.12 53.62,39.5 53.88,39.75 56.12,39.75 56.38,39.5 57.62,39.5 58,39.88 v58.38,39.88
N$58  (via drill 0.4)
  Top 0.254: RN7.3 56.62,34.83 56.62,35.62 57.25,36.25 U23.27 57.25,40.13 v57.12,40.25
  Bottom 0.254: X9.11 23.18,27.05 24.75,28.62 44.62,28.62 47.88,31.88 47.88,33.12 53.12,38.38 53.12,39.75 53.62,40.25 v57.12,40.25
N$59
  Top 0.254: U23.26 56.74,36.49 55.88,35.62 55.88,34.88 RN7.4
N$60
  Top 0.254: X9.12 21.97,29.59 22.55,30.18 RN9.1
N$61
  Top 0.254: RN4.3 77.78,75.22 79.47,73.53 U13.P$5
N$62
  Top 0.254: RN4.4 78.58,75.8 81.67,72.7 U13.P$7
N$63
  Top 0.254: U1.21 98.88,40.72 98.88,39 98.25,38.38 C11.1 R6.1
N$64
  Top 0.406: K5.4 32.62,16.75 32.88,17 R44.1 33.52,18.85 33.12,19.25 33.12,20.23 U27.2 33.9,20.27 34.25,20.62 34.25,24.75 34.75,25.25 36.12,25.25 36.88,26 36.88,28.75 37.02,28.89 U25.6
N$65  (via drill 0.4)
  Top 0.406: C58.1 v35.62,19.25 35.62,18.12 35.23,17.73 R44.2 | v28.12,17 R43.1
  Bottom 0.406: v35.62,19.25 30.5,19.25 v28.12,17
N$66  (via drill 0.4)
  Top 0.406: C57.1 v45.62,19.25 45.62,17.12 45.75,17 R41.1 | v53.5,17 R42.2
  Bottom 0.406: v45.62,19.25 51.25,19.25 v53.5,17
N$67  (via drill 0.4)
  Top 0.254: SJ2.2 v73.75,52.12 | v47.88,34.38 47,35.25 45.5,35.25 44.88,34.62 44.88,31.78 U24.1
  Bottom 0.254: v73.75,52.12 57.38,52.12 51.5,46.12 51.5,38.25 47.88,34.62 v47.88,34.38
N$68  (via drill 0.4)
  Top 0.254: SJ3.2 v73.75,54.62 | v46.25,34 46.25,28.12 45.75,27.62 U24.4
  Bottom 0.254: v73.75,54.62 58.62,54.62 51,47 51,38.75 v46.25,34
N$69  (via drill 0.4)
  Top 0.254: v14,56.25 15.1,56.25 C29.2
  Top 0.305: U15.3 15.29,58.03
  Top 0.406: C29.2 15.15,56.33 15.15,57.9 15.29,58.03
  Top 1.016: v16.25,65.62 R16.1
  Bottom 0.254: 11.72,59.72 11.72,57.41 12.88,56.25 v14,56.25
  Bottom 0.305: K1.1 11.72,59.72
  Bottom 0.406: 11.72,59.72 11.71,59.72
  Bottom 1.016: v16.25,65.62 16.25,63.07 13.14,59.96 11.92,59.96 K1.1
N$70
  Top 0.305: C23.2 71.8,24.95 R12.1
N$71
  Top 0.254: X2.17 35.38,63.01 35.38,60.75 35.88,60.25 38.12,60.25 38.98,59.4 RN2.3
N$77
  Top 0.254: C14.1 116.62,48.12 116.12,47.62 113.65,47.62 U1.49
N$79  (via drill 0.4)
  Top 0.254: X9.7 17.82,27.3 20.75,24.38 23.62,24.38 26.5,27.25 26.5,37.38 27.5,38.38 42.62,38.38 43.75,39.5 43.75,41.62 46.62,44.5 54.75,44.5 U23.14 | RN8.6 19.23,32.48 v17.38,30.62
  Bottom 0.254: v17.38,30.62 17.38,28.17 X9.7
N$80  (via drill 0.4)
  Top 0.254: X9.8 17.43,28.57 21,25 23.5,25 26,27.5 26,37.62 27.25,38.88 42.38,38.88 43.25,39.75 43.25,41.88 46.37,44.99 U23.13 | RN8.5 18.43,32.92 v16.12,30.62
  Bottom 0.254: v16.12,30.62 16.02,30.62 X9.8
N$82
  Top 0.254: U23.34 60.75,36.87 61.62,36 62.44,36 U22.3
N$83
  Top 0.254: U22.1 69.83,30.46 70.25,30.88 R36.1
N$84
  Top 0.305: U14.2 67.49,17.86 67.25,17.62 67.25,16.9 R15.1 67.22,15.53 67.75,15 71.88,15 72.38,15.5 72.38,17.62 71.9,18.1 R13.2
N$87
  Top 0.254: LED1.C R1.2
N$88
  Top 0.406: U25.7 36.7,30.16 36.19,29.77 36.19,26.81 35.5,26.12 32.12,26.12 31,25 31,20.45 U27.1 31.1,20.2 R43.2 31.1,14.65 K5.3
N$89
  Top 0.254: LED7.C 45.38,83.62 45.25,83.5
  Top 1.016: F1.1 42.76,83.5 45.25,83.5 46.55,82.2 SW1.P$3
N$93  (via drill 0.4)
  Top 0.254: U25.1 35.18,31.43 36.25,32.5 36.25,32.75 v37.88,34.38 | v72.25,56.88 72.25,57.88 73.88,59.5 75.12,59.5 SJ4.2
  Bottom 0.254: v37.88,34.38 44.5,34.38 46.38,36.25 47,36.25 50,39.25 50,47.5 58.62,56.12 71.5,56.12 v72.25,56.88
N$94  (via drill 0.4)
  Top 0.254: U25.4 35,27.62 35.5,28.12 35.5,30.62 v37.88,33 | v73.88,56.88 75.12,56.88 SJ5.2
  Bottom 0.254: v37.88,33 43.88,33 46.5,35.62 47.12,35.62 50.5,39 50.5,47.25 58.88,55.62 72.62,55.62 v73.88,56.88
N$95
  Top 1.016: F2.1 44.26,80.87 45.12,80 45.12,73.25 46.33,72.05 SW1.P$1
N$96
  Top 0.254: X2.19 32.88,62.97 32.88,60.38 33.88,59.38 37.62,59.38 38.17,58.83 RN2.4
N$97
  Top 0.254: X2.11 40.58,63.12 RN2.1
N$104
  Top 0.305: R10.2 73.76,22.97 C21.1 | C23.1 C21.1 | C21.1 C24.1
N$105
  Top 0.305: R13.1 73.6,19.11 C24.2
N$106
  Top 0.305: U14.3 68.76,17.14 C26.2
N$109
  Top 0.254: U14.7 67.49,24.86
  Top 0.305: 67.49,24.86 67.49,25.14 67.25,25.38 67,25.38 66.88,25.5 66.9,25.52 R14.2
  Top 0.406: C28.1 63.75,14.12 64.38,14.75 64.38,20.5 65,21.12 66.88,21.12 67.49,21.74 U14.7
N$110
  Top 0.406: C27.2 57.5,11.25 56.5,10.25 56.5,9.12 55.62,8.25 12.75,8.25 11,10 X8.T
N$111
  Top 0.406: C28.2 57.38,14.12 55.62,12.38 55.62,9.25 55.38,9 21.25,9 20,10.25 X8.R
NRST  (via drill 0.4)
  Top 0.2: U6.16 93.6,23.5
  Top 0.254: 92.62,32.88 92.62,35.75 94.49,37.61 94.49,40.64 95,41.15 95,41.78 U1.14 100.12,46.92 100.12,48.38 98.38,50.12 97.25,50.12 96.38,51 v96,51 | 92.62,32.88 92.62,25.75 93.6,24.65 93.6,23.5 | S2.1 56.38,52.15 | 56.38,52.15 68.35,52.15 v69.38,51.12 | 92.62,32.88 92.47,33.02 R3.1 C2.1 | U23.29 58.24,36.76 v58.5,36.5 | v56,49.12 56,51.77 56.38,52.15 | v52.25,39 v52.25,33.62
  Bottom 0.254: v69.38,51.12 84.88,51.12 85.12,50.88 95.88,50.88 v96,51 | S2.1 38,58 38,63.25 36.94,64.31 36.69,64.31 X2.15 | v56,49.12 55.25,49.12 52,45.88 52,39.25 v52.25,39 | v58.5,36.5 58.5,35.62 58.12,35.25 53.25,35.25 52.25,34.25 v52.25,33.62
PA0
  Top 0.2: U6.11 95.6,23.5
  Top 0.254: U1.23 100.12,40.55 100.12,39.38 101,38.5 101.88,38.5 103.62,36.75 103.5,29.12 99.88,25.5 96.38,25.5 95.6,24.73 95.6,23.5
PA1  (via drill 0.4)
  Top 0.2: U6.10 96,23.5
  Top 0.254: U1.24 100.62,40.35 100.62,39.62 101.25,39 102.12,39 104.12,37 104.12,29 100.12,25 96.62,25 96,24.38 96,23.5 | U23.25 56.26,37.01 v55.88,36.62 | U1.24 101.62,41.35 101.62,41.38 102.25,42 v102.25,42.5 | U1.24 101.23,40.98 101.25,41
  Bottom 0.254: v55.88,36.62 55.88,37.75 56.38,38.25 58,38.25 59.12,39.38 59.12,40.12 59.62,40.62 66.75,40.62 68.38,39 71.38,39 76.25,43.88 98.12,43.88 100.12,41.88 101.62,41.88 v102.25,42.5
PA2  (via drill 0.4)
  Top 0.2: U6.9 96.4,23.5
  Top 0.254: 96.4,23.5 96.4,24.02 96.88,24.5 100.38,24.5 104.62,28.75 104.62,37.25 101.59,40.29 U1.25 102.48,41.5 v102.88,41.5 | U23.30 58.75,38.37 58.75,38.38 58.75,39 59,39.25 59.88,39.25 60,39.38 v60,39.88 | 71.47,37.48 v71.5,37.5 71.5,36.62 71.22,36.35 R38.2
  Bottom 0.254: v60,39.88 60.25,40.12 66.5,40.12 68.12,38.5 71.5,38.5 | 71.5,38.5 71.62,38.5 76.5,43.38 97.88,43.38 99.88,41.38 102.75,41.38 v102.88,41.5 | v71.5,37.5 71.5,38.5
PA3
  Top 0.2: U3.16 104.6,23.5
  Top 0.254: 104.25,40.75 U1.26 105.12,39.89 105.12,28.5 104.6,27.98 104.6,23.5
PA4
  Top 0.2: U3.15 105,23.5
  Top 0.254: U1.29 109,38.14 109,31.62 105,27.62 105,23.5
PA5  (via drill 0.4)
  Top 0.2: U3.14 105.4,23.5
  Top 0.254: U1.30 109.5,38.34 109.5,31.12 v105.75,27.38 105.4,27.02 105.4,23.5
  Bottom 0.254: v105.75,27.38 105.75,26.75 102.38,23.38 SJ1.1
PA6
  Top 0.2: U3.13 105.8,23.5
  Top 0.254: U1.31 110,38.55 110,30.5 105.8,26.3 105.8,23.5
PA7  (via drill 0.4)
  Top 0.2: U3.12 106.2,23.5
  Top 0.254: v104.5,43.62 105.62,43.62 106.53,42.72 U1.32 110.5,38.76 110.5,30.25 106.2,25.95 106.2,23.5 | v70.25,39.88 68.75,39.88 67.6,41.02 RN6.1
  Bottom 0.254: v104.5,43.62 104,43.62 103.25,44.38 73,44.38 71.5,42.88 71.5,41.12 v70.25,39.88
PA8
  Top 0.2: U11.4 109.8,77.62
  Top 0.254: U1.67 107.32,57.63 110.25,60.56 110.25,75 109.8,75.45 109.8,77.62
PA9  (via drill 0.4)
  Top 0.2: U11.3 109.4,77.62
  Top 0.203: U1.68 106.89,57.89
  Top 0.254: U18.4 22.21,65.46 v24.12,67.38 24.25,67.5 24.25,68.62 23.96,68.92 R24.1 | v106.75,55.25 106.75,56 106.12,56.62 106.12,57.16 U1.68 109.75,60.79 109.75,74.75 109.4,75.1 109.4,77.62
  Bottom 0.203: v106.75,55.25 106.75,56.12
  Bottom 0.254: 106.75,56.12 96,67.38 94.38,69 25.75,69 v24.12,67.38
PA10  (via drill 0.4)
  Top 0.2: U11.2 109,77.62
  Top 0.203: U1.69 106.53,58.28
  Top 0.254: U18.1 24.14,66.02 v25.75,67.62 26.12,68 26.12,68.62 25.88,68.88 25.15,68.88 R23.1 | v105.62,55.88 105.62,57.37 U1.69 109.25,60.99 109.25,74.5 109,74.75 109,77.62
  Bottom 0.254: v105.62,55.88 93.75,68.5 26.62,68.5 v25.75,67.62
PA11  (via drill 0.4)
  Top 0.2: U11.1 108.6,77.62
  Top 0.203: U1.70 106.13,58.63
  Top 0.254: v104.38,55.5 104.38,56.83 U1.70 108.75,61.2 108.75,74.25 108.6,74.4 108.6,77.62 | R21.1 18.8,43.95 v19.88,42.88
  Bottom 0.254: v104.38,55.5 104.38,56.38 92.75,68 28.25,68 25.62,65.38 25.62,48.62 v19.88,42.88
PA12  (via drill 0.4)
  Top 0.2: U8.8 104.4,77.62
  Top 0.254: v103.38,56.25 103.38,56.53 U1.71 108.25,61.41 108.25,73.5 104.4,77.35 104.4,77.62 | R22.1 18.73,42.39 19.38,41.75 v19.88,41.75
  Bottom 0.254: v103.38,56.25 92.12,67.5 28.5,67.5 26.12,65.12 26.12,48.25 21,43.12 21,42.38 20.38,41.75 v19.88,41.75
PA13  (via drill 0.4)
  Top 0.2: U8.7 104,77.62
  Top 0.203: U1.72 105.34,59.21
  Top 0.254: v104.62,54.25 103.38,54.25 102.5,55.12 102.5,56.75 103.62,57.88 104,57.88 104.25,58.12 U1.72 107.75,61.61 107.75,73.25 104,77 104,77.62 | RN1.3 45.6,63.06 X2.7
  Bottom 0.254: v104.62,54.25 102.38,54.25 90.25,66.5 48.88,66.5 46.91,64.53 46.91,64.36 X2.7
PA14  (via drill 0.4)
  Top 0.2: U8.6 103.6,77.62
  Top 0.254: v101.62,56.75 103.12,58.25 103.12,58.86 U1.76 99.88,62.11 99.88,63.12 103,66.25 103,74.25 103.6,74.85 103.6,77.62 | RN1.4 44.8,59.2 43,61 43,63 X2.9
  Bottom 0.254: v101.62,56.75 101,56.75 90.75,67 46.88,67 44.27,64.39 X2.9
PA15  (via drill 0.4)
  Top 0.2: U8.5 103.2,77.62
  Top 0.254: v100.12,55.38 100.12,56.62 102.25,58.75 102.25,59.03 U1.77 99.38,61.9 99.38,63.38 102.5,66.5 102.5,74.5 103.2,75.2 103.2,77.62 | RN1.2 46.4,59.27 48.12,61 48.12,63.05 X2.5
  Bottom 0.254: v100.12,55.38 100.12,55.62 95.38,60.38 90,66 51.12,66 49.4,64.27 X2.5
PB0  (via drill 0.4)
  Top 0.2: U3.9 107.4,23.5
  Top 0.254: U1.35 112,39.38 112,29.5 110.12,27.62 | 110.12,27.62 107.4,24.9 107.4,23.5 | v110.75,27 110.12,27.62 | R4.1 120.38,27.75 121.25,26.88 v121.25,24.88
  Bottom 0.254: v121.25,24.88 112.88,24.88 v110.75,27
PB1  (via drill 0.4)
  Top 0.2: U5.16 111.6,23.5
  Top 0.254: U1.36 112.5,39.59 112.5,27.38 111.6,26.48 111.6,24.12 | 111.6,23.5 111.6,24.12 | v110.75,24.12 111.6,24.12 | R1.1 123.12,26.62 122.25,25.75 v122.25,24.12
  Bottom 0.254: v122.25,24.12 v110.75,24.12
PB2
  Top 0.2: U5.15 112,23.5
  Top 0.254: U1.37 113,39.79 113,27.12 112,26.12 112,23.5
PB3  (via drill 0.4)
  Top 0.2: U10.1 94.6,77.62
  Top 0.203: U1.89 96.99,55.76
  Top 0.254: v99.75,53.75 99.46,54.04 98.75,54.04 U1.89 93.38,59.42 93.38,74.75 94.6,75.97 94.6,77.62 | X2.13 38,63.08 38,61.25 39.77,59.48 RN2.2
  Bottom 0.254: v99.75,53.75 99.75,54.12 94.38,59.5 41.38,59.5 40.62,60.25 40.62,62.84 40.49,62.97 X2.13
PB4  (via drill 0.4)
  Top 0.2: U7.8 90.4,77.62
  Top 0.203: U1.90 96.67,55.45
  Top 0.254: v98.62,53 98.38,53.25 98.38,53.71 U1.90 92.88,59.21 92.88,74.38 90.4,76.85 90.4,77.62 | RN1.1 47.2,58.95 47.88,59.62 50.38,59.62 50.62,59.88 | 50.62,59.88 50.62,63.01 X2.3 | v54.12,57 54.12,58.75 53.25,59.62 50.88,59.62 50.62,59.88
  Bottom 0.254: v98.62,53 98.62,54.5 94.25,58.88 56,58.88 v54.12,57
PB5  (via drill 0.4)
  Top 0.2: U7.7 90,77.62
  Top 0.254: v98.88,51.5 97.75,52.62 97.75,53.63 U1.91 92.38,59 92.38,74.12 90,76.5 90,77.62 | v77.62,54.62 SJ3.1
  Bottom 0.254: v98.88,51.5 97.75,52.62 97.75,53.5 97.25,54 78.25,54 v77.62,54.62
PB6  (via drill 0.4)
  Top 0.2: U7.6 89.6,77.62
  Top 0.254: v97.62,51 97.62,52 97.25,52.38 97.25,53.42 U1.92 91.88,58.8 91.88,73.88 89.6,76.15 89.6,77.62 | v77.62,52.12 SJ2.1
  Bottom 0.254: v97.62,51 97.62,51.88 97.25,52.25 97.25,53.12 96.88,53.5 79,53.5 v77.62,52.12
PB7  (via drill 0.4)
  Top 0.2: U7.5 89.2,77.62
  Top 0.254: 92.73,57.23 91.38,58.59 91.38,73.62 89.2,75.8 89.2,77.62 | 92.73,57.23 U1.93 | 37.5,42.88 36.5,42.88 35.77,42.15 R2.1 C1.1 | 37.5,42.88 43.5,42.88 46.25,45.62 47.38,45.62 v48.25,46.5 | v92.62,56.88 92.62,57.12 92.73,57.23 | S1.1 36.73,52.15 37.5,51.38 37.5,42.88
  Bottom 0.254: v48.25,46.5 60.12,58.38 91.12,58.38 v92.62,56.88
PB8  (via drill 0.4)
  Top 0.2: U7.4 88.8,77.62
  Top 0.254: U1.95 93.3,55.25 92.88,55.25 v91.25,56.88 90.88,57.25 90.88,73.38 88.8,75.45 88.8,77.62 | v82.12,56.88 76.38,56.88 SJ5.1
  Bottom 0.254: v91.25,56.88 v82.12,56.88
PB9  (via drill 0.4)
  Top 0.2: U7.3 88.4,77.62
  Top 0.254: U1.96 93.09,54.75 92,54.75 v91,55.75 90.38,56.38 90.38,73.12 88.4,75.1 88.4,77.62 | SJ4.1 81.62,59.38 v85.25,55.75
  Bottom 0.254: v85.25,55.75 v91,55.75
PB10
  Top 0.2: U4.13 119.8,23.5
  Top 0.254: U1.47 118,41.88 118,27.62 119.8,25.82 119.8,23.5
PB11  (via drill 0.4)
  Top 0.2: U4.12 120.2,23.5
  Top 0.254: v66.62,48.25 66.12,48.25 65.41,48.97 RN5.1 | v109.38,48.12 110.38,49.12 111.5,49.12 112.19,48.43 U1.48 118.5,42.12 118.5,27.88 120.2,26.18 120.2,23.5
  Bottom 0.254: v66.62,48.25 67.62,49.25 108.38,49.25 109.38,48.25 v109.38,48.12
PB12  (via drill 0.4)
  Top 0.254: v109.62,50.5 109.88,50.75 111.75,50.75 U1.51 112.91,51.91 118.25,57.25 118.25,71.25 123.8,76.8 U12.4 | v66.62,49.5 65.88,49.5 65.61,49.77 RN5.2
  Bottom 0.254: v109.62,50.5 108.88,49.75 66.88,49.75 v66.62,49.5
PB13  (via drill 0.4)
  Top 0.254: v108.62,51.25 111.5,51.25 112.52,52.27 U1.52 112.55,52.3 117.75,57.5 117.75,71.5 123.4,77.15 U12.3 | v66.62,50.75 66.12,50.75 65.94,50.57 RN5.3
  Bottom 0.254: v108.62,51.25 107.62,50.25 67.12,50.25 v66.62,50.75
PB14
  Top 0.254: U12.2 123,77.5 117.25,71.75 117.25,57.69 U1.53
PB15
  Top 0.254: U1.54 116.75,57.88 116.75,72 122.6,77.85 U12.1
PC0
  Top 0.2: U6.15 94,23.5
  Top 0.254: U1.15 95.5,41.59 95.5,40.88 95,40.38 95,37.38 93.12,35.5 93.12,26.12 94,25.25 94,23.5
PC1  (via drill 0.4)
  Top 0.2: U6.14 94.4,23.5
  Top 0.254: U1.16 96.01,41.39 96.01,40.51 95.5,40.01 95.5,37.12 93.62,35.25 93.62,28.5 94.4,27.73 94.4,26.88 | 94.4,23.5 94.4,26.88 | U23.31 59.25,36.13 58.88,35.38 v58.88,32.25 | v58.88,30.75 v60.88,28.75 | v93.88,26.88 94.4,26.88
  Bottom 0.254: v58.88,32.25 v58.88,30.75 | v60.88,28.75 61.25,28.38 85.88,28.38 87.38,26.88 v93.88,26.88
PC2  (via drill 0.4)
  Top 0.2: U6.13 94.8,23.5
  Top 0.254: v97.01,39.23 97.01,39.51 96.65,39.88 96.65,41.32 U1.17 | 94.8,23.5 94.8,25.43 v96.12,26.75
  Bottom 0.254: v97.01,39.23 96.12,38.35 v96.12,26.75 96.11,27.73
PC3  (via drill 0.4)
  Top 0.2: U6.12 95.2,23.5
  Top 0.254: v97.5,40.38 97.5,41.46 U1.18 | 95.2,23.5 95.2,25.07 96.12,26 96.5,26 v97.25,26.75
  Bottom 0.254: v97.25,26.75 97.25,38.25 97.88,38.88 97.88,40 v97.5,40.38
PC4  (via drill 0.4)
  Top 0.2: U3.11 106.6,23.5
